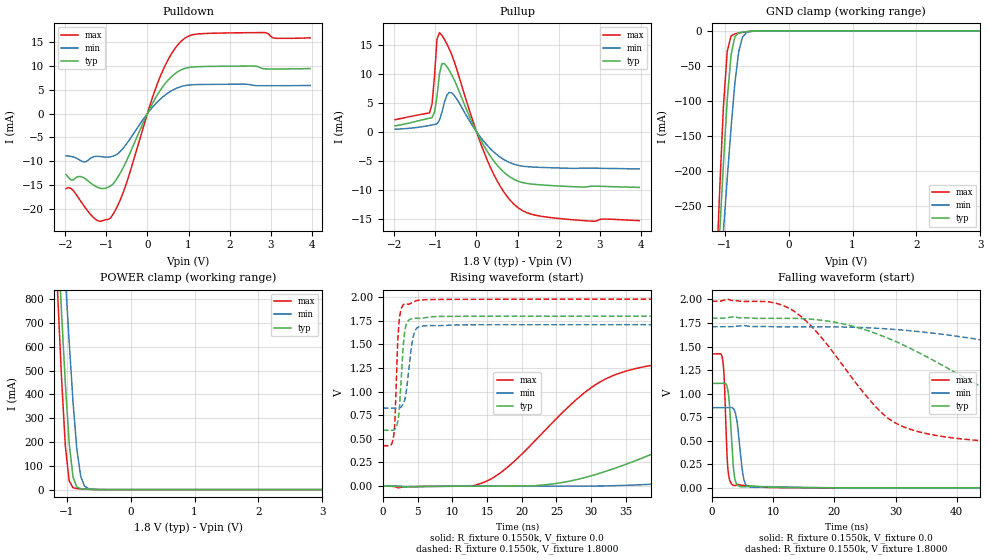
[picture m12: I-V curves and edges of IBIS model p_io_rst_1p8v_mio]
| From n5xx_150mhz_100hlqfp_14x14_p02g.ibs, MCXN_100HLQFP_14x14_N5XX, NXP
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[Model] p_io_rst_1p8v_mio
|   Model p_io_rst_1p8v_mio
| This model was characterised for following simulation conditions:
| External (pad) voltage:
|   - Typ: 1.8V,   - Min: 1.71V,   - Max: 1.98V
| Library cells for typ/min/max conditions are connected as defined below:
|  pad - External Pad
|  ipp_do_lv - Core Input
|  ipp_obe_lv - Output Buffer Enable
|  IOGC - NC
|  REFH3V3 - REFH3V3
|  REFL3V3 - REFL3V3
|  ZI - NC
|  abut_ncal_vddio[1] - vssio vddio vddio
|  abut_ncal_vddio[2] - vddio vddio vssio
|  abut_ncal_vddio[3] - vddio
|  abut_ncal_vddio[4] - vssio vddio vddio
|  abut_ncal_vddio[5] - vddio vddio vssio
|  abut_ncal_vddio[6] - vddio
|  abut_pcal_vddio[1] - vssio
|  abut_pcal_vddio[2] - vddio vssio vddio
|  abut_pcal_vddio[3] - vssio
|  abut_pcal_vddio[4] - vssio
|  abut_pcal_vddio[5] - vddio vssio vddio
|  abut_pcal_vddio[6] - vssio
|  ipp_do_1p8v - ipp_do_1p8v
|  ipp_eftd_lv - NC
|  ipp_ina_mux_vddio - NC
|  ipp_ina_mux_vddio[0] - NC
|  ipp_ina_mux_vddio[1] - NC
|  ipp_ina_r0_vddio - NC
|  ipp_ina_r0a_vddio - NC
|  ipp_ina_r0b_vddio - NC
|  ipp_ina_r0c_vddio - NC
|  ipp_ina_r0d_vddio - NC
|  ipp_ina_r0e_vddio - NC
|  ipp_ina_r0f_vddio - NC
|  ipp_ina_r300_vddio - NC
|  ipp_ina_r300a_vddio - NC
|  ipp_ina_r300b_vddio - NC
|  ipp_ina_r300c_vddio - NC
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Model_type I/O
Polarity   Non-Inverting
Enable   Active-High
Vinl =   0.5400V
Vinh =   1.2600V
Vmeas =  0.9000V
Cref =   30.0000pF
Rref =   1.0000M
Vref =   1.8000V
C_comp   1.3080pF   1.2614pF   1.4172pF
|C_comp_pullup   0.5655pF   0.5989pF   0.5406pF
|C_comp_pulldown   0.6531pF   0.7268pF   0.6283pF
[Model Spec]
| variable   typ   min   max
Vinh   1.2600V   1.1970V   1.3860V
Vinl   0.5400V   0.5130V   0.5940V
[Temperature Range]   25.0000   0.1250k   -40.0000
[Voltage Range]   1.8000V   1.7100V   1.9800V
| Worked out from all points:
|   slope of the pulldown table from 0 to 0.27 V, typ, clamps not added: 62.4 ohm
|   slope of the pullup table from 0 to 0.27 V, typ, clamps not added: 77.5 ohm
|   GND clamp passes 1 mA (typ) near -0.64 V on its own axis
|   POWER clamp passes 1 mA (typ) near -0.63 V on its own axis
|   rising waveform, R_fixture 0.1550k, V_fixture 0.0: 20-80 % time 25.4ns typ, 47ns min, 12.9ns max; typ from 0 V to 1.11 V
|   rising waveform, R_fixture 0.1550k, V_fixture 1.8000: 20-80 % time 632ps typ, 878ps min, 492ps max; typ from 0.592 V to 1.8 V
|   falling waveform, R_fixture 0.1550k, V_fixture 0.0: 20-80 % time 639ps typ, 845ps min, 495ps max; typ from 1.11 V to 0 V
|   falling waveform, R_fixture 0.1550k, V_fixture 1.8000: 20-80 % time 23.6ns typ, 44.8ns min, 11.9ns max; typ from 1.8 V to 0.592 V
[Pulldown]
|Voltage   I(typ)   I(min)   I(max)
-1.98V    -12.82mA   -8.883mA   -15.79mA
-1.8V     -13.92mA   -9.12mA    -16.22mA
-1.56V    -13.44mA   -10.16mA   -19.21mA
-1.26V    -15.3mA    -8.987mA   -22.25mA
-900mV    -15.23mA   -9.092mA   -21.98mA
-540mV    -10.5mA    -6.733mA   -15.41mA
300mV     4.734mA    2.929mA    7.544mA
600mV     7.861mA    4.866mA    12.77mA
960mV     9.609mA    5.948mA    16.11mA
2.82V     9.429mA    5.854mA    17.02mA
3.12V     9.374mA    5.856mA    15.82mA
3.96V     9.46mA     5.905mA    15.92mA
[Pullup]
|Voltage   I(typ)   I(min)   I(max)
-1.98V    969uA      399.5uA    2.039mA
-1.14V    2.305mA    1.059mA    3.215mA
-1.08V    2.398mA    1.144mA    4.758mA
-1.02V    3.354mA    1.233mA    9.535mA
-960mV    6.027mA    1.324mA    15.88mA
-900mV    9.906mA    1.971mA    17.06mA
-780mV    11.71mA    5.028mA    15.89mA
-600mV    9.758mA    6.666mA    13.21mA
240mV     -3.146mA   -2.189mA   -4.533mA
900mV     -8.184mA   -5.592mA   -12.42mA
1.68V     -9.239mA   -6.201mA   -14.7mA
3.96V     -9.621mA   -6.444mA   -15.35mA
[GND_clamp]
|Voltage   I(typ)   I(min)   I(max)
-1.98V    -2.029A    -1.716A    -2.516A
-1.14V    -399.2mA   -446.6mA   -369.9mA
-1.08V    -292.8mA   -366.2mA   -232.1mA
-1.02V    -191mA     -287.4mA   -109mA
-960mV    -98.91mA   -211.2mA   -29.36mA
-900mV    -34.26mA   -138.9mA   -7.283mA
-840mV    -8.248mA   -74.31mA   -4.319mA
-780mV    -2.995mA   -29.56mA   -3.112mA
-720mV    -1.791mA   -8.837mA   -2.149mA
-660mV    -1.158mA   -2.642mA   -1.361mA
-600mV    -697.2uA   -1.05mA    -760.6uA
3.96V     0A         0A         0A
[POWER_clamp]
|Voltage   I(typ)   I(min)   I(max)
-1.98V    5.575A     5.314A     6.031A
-1.14V    1.063A     1.433A     822.6mA
-1.08V    748.7mA    1.161A     472.7mA
-1.02V    446mA      889.8mA    183.6mA
-960mV    194.9mA    621.5mA    36.74mA
-900mV    52.34mA    369.1mA    7.81mA
-840mV    10.74mA    169.6mA    4.436mA
-780mV    3.619mA    56.13mA    3.182mA
-720mV    2.073mA    15.03mA    2.194mA
-660mV    1.305mA    4.298mA    1.374mA
-360mV    5.031uA    27.49uA    1.319uA
3.96V     0A         0A         0A
[Ramp]
| variable   typ   min   max
dV/dt_r  0.6651/25.3831n   0.5064/47.0628n   0.8531/12.9182n
dV/dt_f  0.7248/23.6086n   0.5259/44.8225n   0.9321/11.9089n
R_load = 0.1550k
[Rising Waveform]
R_fixture= 0.1550k
V_fixture= 0.0
V_fixture_min= 0.0
V_fixture_max= 0.0
|time   V(typ)   V(min)   V(max)
0s        394pV      138.2nV    9.262pV
14.46ns   -1.261mV   -1.191mV   36.97mV
18.4ns    -509.8uV   -887.1uV   227.7mV
31.3ns    136.9mV    580.7uV    1.104V
45.84ns   556.9mV    62.66mV    1.342V
56.06ns   822.9mV    161mV      1.384V
66.29ns   953mV      285.5mV    1.403V
91.05ns   1.059V     583.6mV    1.418V
111.1ns   1.087V     710.6mV    1.421V
231.3ns   1.109V     844mV      1.422V
[Rising Waveform]
R_fixture= 0.1550k
V_fixture= 1.8000
V_fixture_min= 1.7100
V_fixture_max= 1.9800
|time   V(typ)   V(min)   V(max)
0s        591.7mV    826.7mV    426.4mV
1.57ns    591.7mV    826.7mV    535.5mV
1.753ns   603.9mV    826.7mV    716.8mV
2.198ns   703.2mV    824.3mV    1.604V
2.6ns     1.079V     836.4mV    1.867V
2.975ns   1.52V      878.7mV    1.923V
3.358ns   1.708V     994.7mV    1.931V
4.373ns   1.776V     1.579V     1.95V
5.43ns    1.775V     1.692V     1.971V
231.3ns   1.8V       1.71V      1.98V
[Falling Waveform]
R_fixture= 0.1550k
V_fixture= 0.0
V_fixture_min= 0.0
V_fixture_max= 0.0
|time   V(typ)   V(min)   V(max)
0s        1.109V     850.6mV    1.422V
1.78ns    1.109V     850.6mV    1.353V
2.022ns   1.11V      850.7mV    1.155V
2.521ns   1.065V     850.6mV    293.1mV
2.878ns   880.8mV    851.1mV    88.96mV
3.698ns   116.2mV    819mV      24.33mV
4.128ns   34.09mV    697mV      34.73mV
5.249ns   11.03mV    84.39mV    25.45mV
6.651ns   18.71mV    6.021mV    14.43mV
231.3ns   250.1nV    3.587uV    12.7nV
[Falling Waveform]
R_fixture= 0.1550k
V_fixture= 1.8000
V_fixture_min= 1.7100
V_fixture_max= 1.9800
|time   V(typ)   V(min)   V(max)
0s        1.8V       1.71V      1.98V
12.47ns   1.8V       1.709V     1.911V
16.89ns   1.786V     1.71V      1.671V
28.7ns    1.59V      1.687V     743.2mV
41.67ns   1.156V     1.594V     513.4mV
49.78ns   903.4mV    1.505V     476.2mV
59.8ns    758.8mV    1.369V     453.3mV
80.87ns   657.1mV    1.092V     434.6mV
100.4ns   622.9mV    968.8mV    429.3mV
231.3ns   592.1mV    833.5mV    426.4mV
